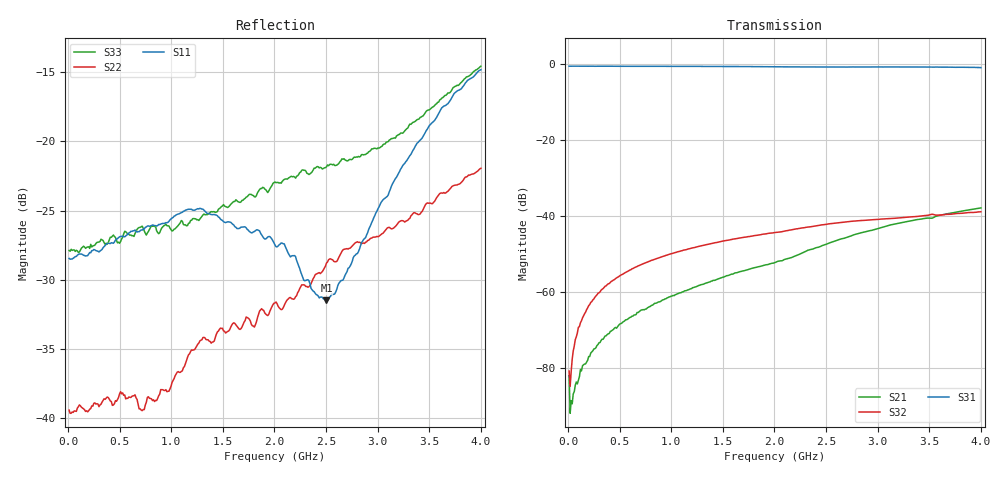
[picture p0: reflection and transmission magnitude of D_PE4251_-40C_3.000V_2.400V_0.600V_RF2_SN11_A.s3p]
! Device ID: PE4251_SoldCshunt_081809
! Dir: c:\Test Bench Repositories\Bench_Software_CVI_Version_8\trunk\PSC 4Port_VNA Bench\datalog\4250\TEST\PE4251_SoldCshunt_081809\-40C\3p000000\RF2
! Serial: 11
! Insertion: A
! Temp: -40C
! VDD: 3.000
! Control_Hi: 80.000
! Control_Lo: 20.000
! Logic State: RF2
! Port 1: RFC
! Port 2: RF1
! Port 3: RF2
! V1 = 0.60
! V2 = 0.60
! V3 = 0.60
! IDD: 4.129990e-05
! FILE NAME
! DATE 08/18/09  20:08
! CORRECTED  DATA
#  Hz  S  RI  R  50.00
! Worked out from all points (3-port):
!   401 points, 10 MHz to 4 GHz, reference 50 ohm
!   strongest paths, dB at 10 MHz, 1.008 GHz, 2.005 GHz, 3.002 GHz, 4 GHz:
!     S31: -0.5, -0.5, -0.6, -0.7, -0.9
!     S32: -80.8, -49.8, -44.3, -40.9, -38.8
!     S21: -82.0, -61.0, -52.2, -43.3, -37.8
!   lowest |S11| = -31.5 dB at 2.504 GHz (marker M1), VSWR 1.05, Z = 50.6 - j2.61 ohm
!   |S11| at or under -10 dB: start of sweep to end of sweep
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1e7  0.0378 -0.000611  -2.15e-05 -3.45e-05  0.9451 -0.00334
     6.89e-05 3.92e-05  0.0107 -0.000653  1.31e-05 -3.87e-05
     0.9452 -0.00403  -1.72e-05 8.95e-05  0.0403 0.000703
9.9775e7  0.039 0.00201  7.95e-06 -7.94e-05  0.9442 -0.0356
          8.27e-06 -6.82e-05  0.011 0.000471  3.23e-05 0.000328
          0.9452 -0.0359  3.27e-05 0.000341  0.0397 2.36e-06
1.79575e8  0.0385 0.00335  -1.41e-05 -0.000123  0.9427 -0.0625
           -1.6e-05 -0.000119  0.0106 0.00127  4.42e-05 0.000585
           0.9425 -0.0631  4.75e-05 0.000585  0.0414 0.000727
4.888e8  0.0446 0.00528  -0.000186 -0.000312  0.9273 -0.168
         -0.000181 -0.000315  0.0116 0.00271  0.000149 0.0016
         0.928 -0.1677  0.000139 0.00158  0.0431 -0.00261
7.18225e8  0.0477 0.00209  -0.000392 -0.000421  0.9098 -0.2437
           -0.000394 -0.000428  0.00997 0.00374  0.000281 0.00231
           0.9111 -0.2435  0.000281 0.00232  0.0491 -0.00555
1.276825e9  0.0567 -0.00867  -0.0011 -0.000541  0.8391 -0.4183
            -0.0011 -0.000553  0.0173 0.00795  0.000688 0.00397
            0.8411 -0.4178  0.000684 0.00397  0.0516 -0.00883
2.005e9  0.0382 -0.0181  -0.00233 -0.000753  0.7028 -0.6057
         -0.00233 -0.00075  0.0165 0.0202  0.00125 0.00595
         0.7043 -0.606  0.00124 0.00596  0.0654 -0.0283
2.50375e9  0.00641 -0.0258  -0.00409 -0.00124  0.5927 -0.7045
           -0.0041 -0.00124  0.0186 0.0312  0.00173 0.00762
           0.5954 -0.7044  0.00173 0.00761  0.0531 -0.061
3.371575e9  -0.0894 -0.0376  -0.00895 0.000214  0.3613 -0.8475
            -0.00896 0.000231  -0.00101 0.0548  0.00265 0.00952
            0.3633 -0.8489  0.00262 0.00953  -0.0181 -0.1174
4e9  -0.1799 -0.0227  -0.0126 0.00258  0.1411 -0.8959
     -0.0126 0.00256  -0.03 0.0741  0.00284 0.011
     0.1419 -0.8951  0.00283 0.0111  -0.1275 -0.1365
